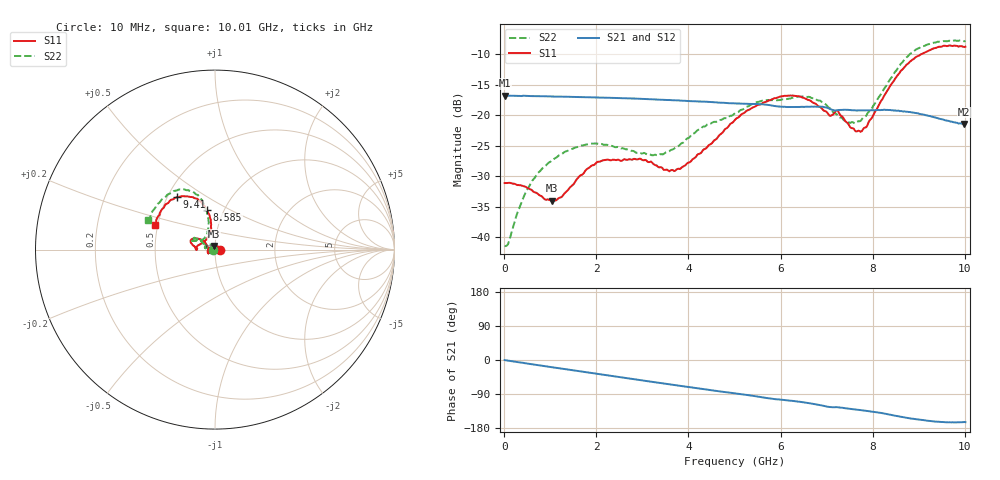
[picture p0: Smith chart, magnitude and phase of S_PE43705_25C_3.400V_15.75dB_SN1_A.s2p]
! Device ID: PE43705
! Serial: 1
! Insertion: A
! Impedance: 50 ohm
! Temp: 25C
! VDD: 3.400V
! Attenuation Step: 15.75dB
#  Hz  S  RI  R  50
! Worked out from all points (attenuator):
!   401 points, 10 MHz to 10.01 GHz, reference 50 ohm
!   highest |S21| = -16.77 dB at 10 MHz (marker M1); lowest = -21.4 dB at 9.985 GHz (marker M2)
!   lowest |S11| = -34.0 dB at 1.035 GHz (marker M3), VSWR 1.04, Z = 49.6 + j1.95 ohm
!   |S11| at or under -10 dB: start of sweep to 9.053 GHz
!   |S22| runs from -41.4 to -7.8 dB; largest |S21 - S12| = 0.0014
!   S11 on the Smith chart (normalised r, x): 10 MHz: 1.06, +0.00; 8.585 GHz: 0.83, +0.38; 9.41 GHz: 0.56, +0.37; 10.01 GHz: 0.48, +0.15
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1e7  0.0278 0.00023  0.145 -0.000657  0.145 -0.000582  -0.00853 0.000522
1.1e8  0.0278 0.00349  0.1444 -0.00533  0.1443 -0.00529  -0.00784 0.00522
5.35e8  0.0185 0.0169  0.1415 -0.025  0.1415 -0.0248  -0.0142 0.0217
1.035e9  -0.00397 0.0196  0.1347 -0.0465  0.1347 -0.0463  -0.0317 0.0285
1.685e9  -0.0321 0.00517  0.1212 -0.0715  0.1213 -0.0715  -0.0525 0.021
2.21e9  -0.0415 -0.0121  0.1068 -0.0892  0.1068 -0.0892  -0.0565 0.0104
2.96e9  -0.0385 -0.0212  0.0814 -0.1093  0.0816 -0.1091  -0.0481 0.00966
3.36e9  -0.034 -0.0157  0.0666 -0.1166  0.0667 -0.1164  -0.0455 0.0126
3.86e9  -0.0373 0.00439  0.0474 -0.1228  0.0475 -0.1226  -0.0538 0.0248
5.01e9  -0.074 0.0543  0.00409 -0.125  0.00432 -0.125  -0.0886 0.0544
5.985e9  -0.1294 0.0585  -0.0295 -0.1139  -0.0289 -0.114  -0.118 0.0615
6.685e9  -0.1254 0.0264  -0.0502 -0.1062  -0.0501 -0.1063  -0.128 0.0512
7.06e9  -0.0991 0.00629  -0.0632 -0.0935  -0.0631 -0.0941  -0.1027 0.0507
7.235e9  -0.1083 0.0116  -0.0625 -0.0905  -0.0622 -0.0905  -0.0878 0.0485
7.435e9  -0.0816 0.031  -0.0678 -0.0874  -0.0676 -0.0876  -0.0704 0.0563
7.71e9  -0.0514 0.0539  -0.073 -0.0817  -0.0727 -0.0816  -0.0522 0.0723
8.36e9  -0.024 0.1678  -0.0893 -0.0651  -0.0892 -0.0653  -0.0405 0.1887
8.585e9  -0.0447 0.2186  -0.093 -0.0548  -0.0924 -0.0557  -0.0596 0.2484
8.935e9  -0.0974 0.2828  -0.0954 -0.042  -0.0953 -0.0416  -0.1231 0.3219
9.41e9  -0.2128 0.2916  -0.0903 -0.028  -0.0901 -0.0277  -0.2316 0.3257
9.985e9  -0.329 0.1487  -0.0815 -0.024  -0.082 -0.0238  -0.3626 0.1764
1.001e10  -0.3363 0.1397  -0.0821 -0.0236  -0.0821 -0.0242  -0.3709 0.1652
